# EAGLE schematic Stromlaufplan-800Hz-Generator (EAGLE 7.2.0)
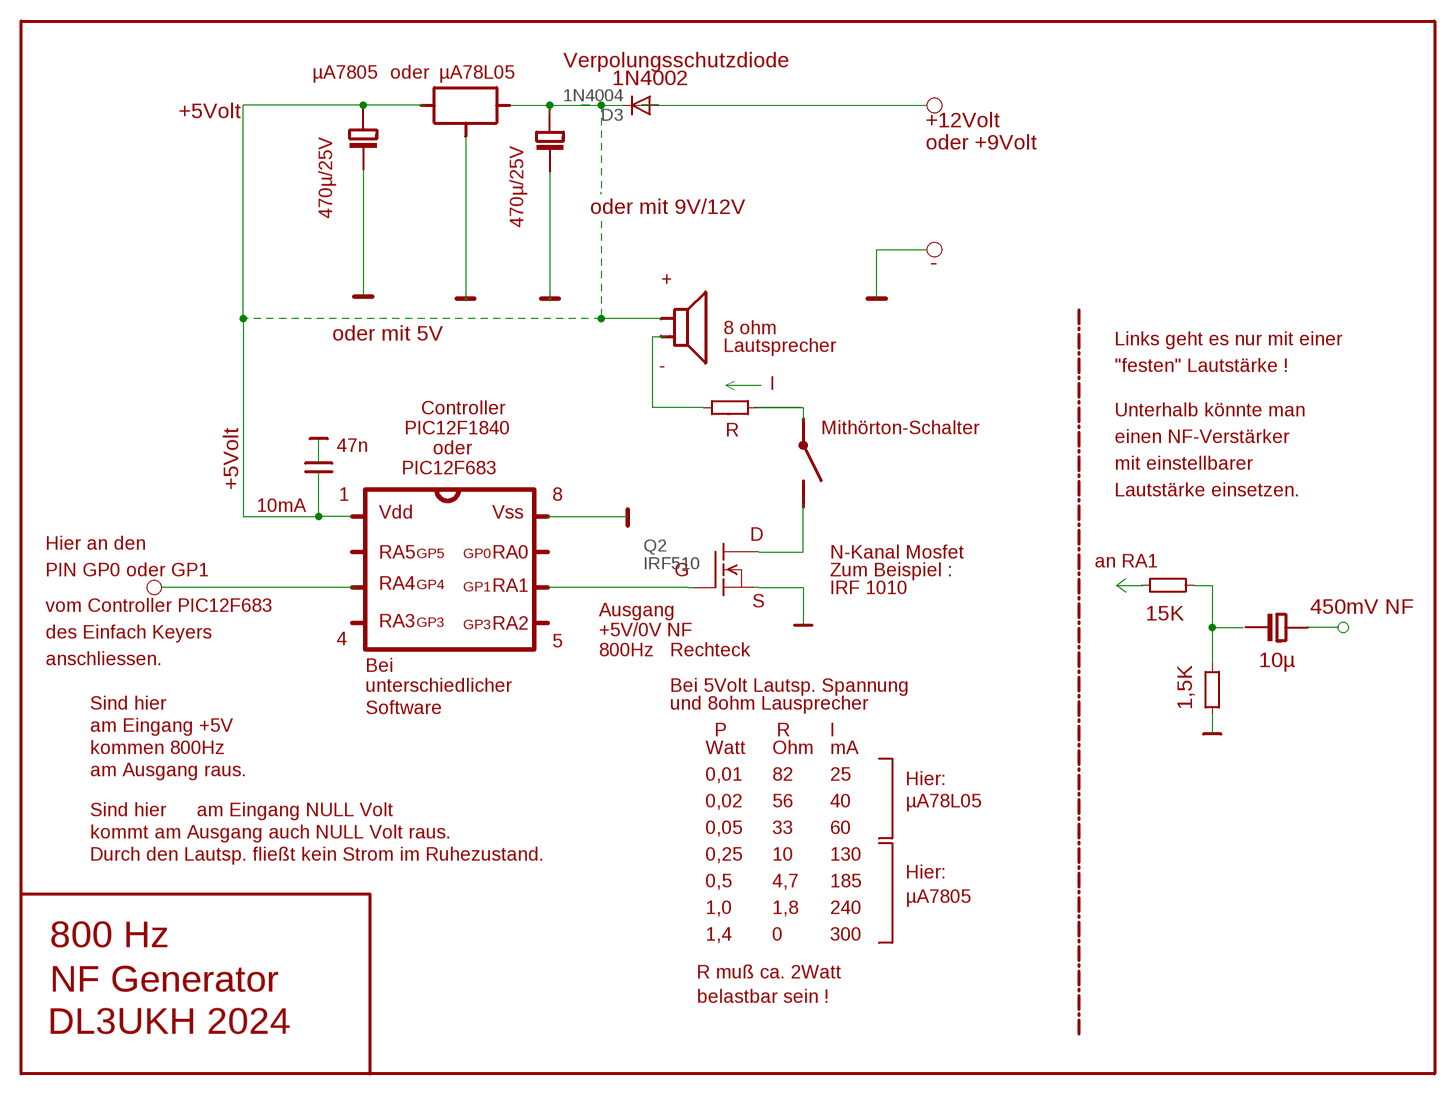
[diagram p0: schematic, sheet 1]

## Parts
D3  1N4004  [DO41-10]
Q2  IRF510  [TO220]

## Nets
N$8: D3.C
N$47: D3.A
N$55: Q2.1(G)
N$71: Q2.3(S)
N$76: Q2.2(D)

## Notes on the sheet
- Verpolungsschutzdiode
- µA7805 | oder | µA78L05
- 1N4002
- +5Volt
- +12Volt
- oder +9Volt
- 470µ/25V | oder mit 9V/12V
- 470µ/25V
- -
- +
- 8 ohm
- oder mit 5V | Links geht es nur mit einer
- Lautsprecher
- - | "festen" Lautstärke !
- I
- Controller
- PIC12F1840 | Unterhalb könnte man
- +5Volt
- R | Mithörton-Schalter
- oder | einen NF-Verstärker
- 47n
- PIC12F683
- mit einstellbarer
- 1 | 8 | Lautstärke einsetzen.
- 10mA
- Vdd | Vss
- D
- Hier an den
- RA5 | GP5 | GP0 | RA0 | N-Kanal Mosfet
- an RA1
- PIN GP0 oder GP1 | G | Zum Beispiel :
- RA4 | GP4 | GP1 | RA1 | IRF 1010
- vom Controller PIC12F683 | S
- Ausgang | 450mV NF
- 15K
- RA3 | GP3 | GP3 | RA2
- des Einfach Keyers | +5V/0V NF
- 4 | 5
- 800Hz | Rechteck
- anschliessen. | 10µ
- Bei
- unterschiedlicher | Bei 5Volt Lautsp. Spannung
- Sind hier | Software | und 8ohm Lausprecher | 1,5K
- am Eingang +5V | P | R | I
- kommen 800Hz | Watt | Ohm | mA
- am Ausgang raus. | 0,01 | 82 | 25
- Hier:
- 0,02 | 56 | 40 | µA78L05
- Sind hier | am Eingang NULL Volt
- kommt | am Ausgang auch NULL Volt raus. | 0,05 | 33 | 60
- Durch den Lautsp. fließt kein Strom im Ruhezustand. | 0,25 | 10 | 130
- Hier:
- 0,5 | 4,7 | 185
- µA7805
- 1,0 | 1,8 | 240
- 1,4 | 0 | 300
- 800 Hz
- R muß ca. 2Watt
- NF Generator
- belastbar sein !
- DL3UKH 2024

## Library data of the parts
D3 = diode:1N4004: DIODE
Q2 = transistor-fet:IRF510: N-Channel Enhancement MOSFET (HEXFET); 100V; 5,6A; 0,54Ohm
